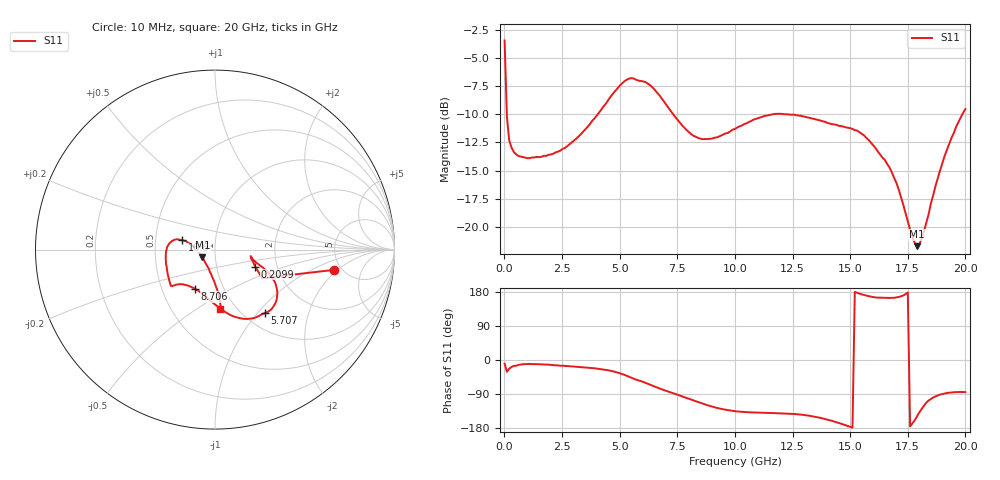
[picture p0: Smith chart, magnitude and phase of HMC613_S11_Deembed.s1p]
!Agilent Technologies,N5224A,MY51441113,A.09.90.11
!Agilent N5224A: A.09.90.11
!Date: Monday, July 24, 2017 14:22:38
!Correction: S11(Full 1 Port(1))
!S1P File: Measurement: S11:
# Hz S  dB  R 50
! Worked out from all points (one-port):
!   201 points, 10 MHz to 20 GHz, reference 50 ohm
!   lowest |S11| = -21.7 dB at 17.9 GHz (marker M1), VSWR 1.18, Z = 43.3 - j3.72 ohm
!   |S11| at or under -10 dB: 106.6 MHz to 4.052 GHz (3.945 GHz wide, 190 % of centre); 7.323 GHz to 11.65 GHz (4.33 GHz wide, 45.6 % of centre); 12.24 GHz to 19.87 GHz (7.628 GHz wide, 47.5 % of centre)
!   S11 on the Smith chart (normalised r, x): 10 MHz: 4.31, -1.78; 209.9 MHz: 1.54, -0.31; 5.707 GHz: 1.24, -1.10; 8.706 GHz: 0.73, -0.34; 16.6 GHz: 0.69, +0.07; 20 GHz: 0.85, -0.63
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1e7  -3.46 -9.7
1.0995e8  -10.23 -31.1
2.099e8  -12.31 -22.9
4.098e8  -13.35 -15.5
1.0095e9  -13.89 -10.6
2.50875e9  -13.09 -15.1
3.30835e9  -11.79 -18.7
4.10795e9  -9.86 -23.3
5.0075e9  -7.46 -34.9
5.30735e9  -6.94 -41.6
5.70715e9  -6.94 -51.7
6.4068e9  -7.58 -67.5
7.50625e9  -10.48 -91.5
8.2059e9  -11.91 -106.7
8.70565e9  -12.19 -117.1
1.0005e10  -11.30 -135.1
1.130435e10  -10.14 -139.4
1.250375e10  -10.03 -142.2
1.36032e10  -10.50 -151.2
1.50025e10  -11.23 -176.3
1.58021e10  -12.27 168.4
1.66017e10  -14.38 164.0
1.70015e10  -16.05 165.1
1.750125e10  -19.50 178.2
1.790105e10  -21.68 -148.8
1.82009e10  -20.38 -120.6
1.910045e10  -13.68 -88.4
2e10  -9.53 -84.8
